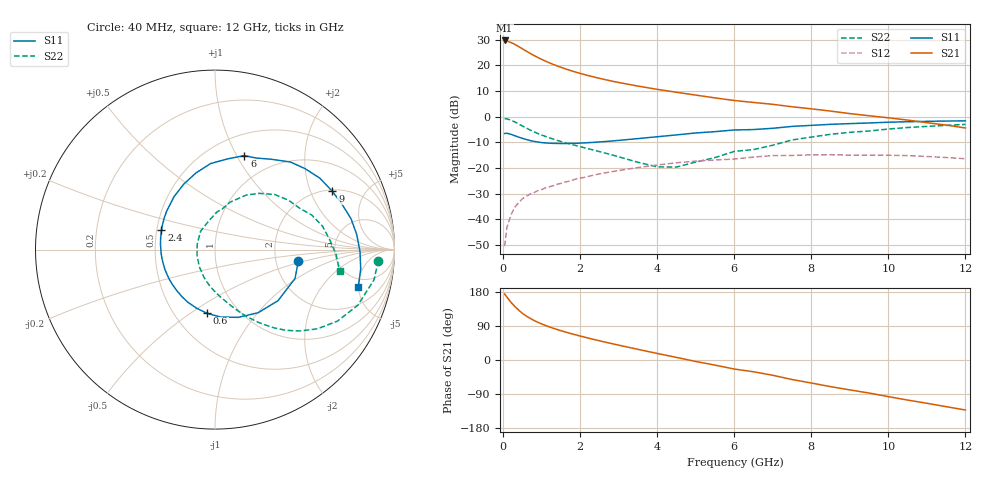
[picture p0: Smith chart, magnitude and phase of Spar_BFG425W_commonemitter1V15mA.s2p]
! Filename: 115bfg425.001
! BFG425W Field C1
! V1=8.654E-001V,V2=1.000E+000V, I1=2.240E-004A, I2=1.501E-002A
# GHz  S  MA  R 50
!  S11  S21  S12  S22
!Freq(GHz)  Mag  Ang  Mag  Ang  Mag  Ang  Mag  Ang
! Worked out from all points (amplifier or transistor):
!   44 points, 40 MHz to 12 GHz, reference 50 ohm
!   highest |S21| = 29.6 dB at 40 MHz (marker M1)
!   |S21| within 3 dB of that: start of sweep to 474.3 MHz
!   unconditionally stable (mu >= 1): 1.434 GHz to end of sweep
!   at 700 MHz: K = 0.69, MSG = 27.4 dB, |S12| = -30.2 dB
!   at 2.4 GHz: K = 1.15, MAG = 16.6 dB, |S12| = -22.6 dB
!   at 12 GHz: K = 1.36, MAG = 2.4 dB, |S12| = -16.4 dB
!   S11 on the Smith chart (normalised r, x): 40 MHz: 2.68, -0.44; 600 MHz: 0.72, -0.58; 2.4 GHz: 0.53, +0.13; 6 GHz: 0.72, +1.08; 9 GHz: 2.07, +2.88; 12 GHz: 3.84, -4.97
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0.04  0.469 -7.9  30.36 174.1  0.003 76.3  0.912 -3.9
0.1  0.474 -19.8  29.61 166.0  0.007 81.6  0.902 -10.7
0.2  0.452 -39.0  27.79 152.8  0.012 74.0  0.854 -21.3
0.3  0.426 -55.7  25.61 141.8  0.017 68.6  0.79 -30.3
0.4  0.399 -71.1  23.21 131.9  0.021 63.9  0.722 -37.7
0.5  0.377 -85.2  20.93 123.3  0.025 60.3  0.657 -43.6
0.6  0.358 -97.0  18.87 116.2  0.028 57.9  0.6 -48.6
0.7  0.342 -107.6  17.07 110.1  0.031 55.9  0.549 -52.7
0.9  0.32 -125.5  14.19 99.6  0.036 53.4  0.47 -59.3
1  0.312 -133.2  13.03 95.2  0.038 52.5  0.438 -62.1
1.2  0.304 -146.4  11.16 87.4  0.043 50.8  0.387 -67.1
1.6  0.299 -168.0  8.59 74.4  0.053 47.8  0.312 -75.8
2.2  0.31 167.4  6.316 58.2  0.068 42.0  0.238 -89.3
2.4  0.317 160.3  5.793 53.2  0.074 39.9  0.218 -94.2
3.5  0.373 127.8  3.924 28.1  0.102 25.5  0.129 -132.9
4.5  0.44 104.0  2.976 6.8  0.126 10.5  0.104 162.0
6  0.549 72.7  2.057 -23.8  0.149 -13.9  0.21 87.0
6.5  0.559 65.8  1.886 -31.0  0.163 -17.8  0.228 80.2
8.5  0.707 34.2  1.28 -70.3  0.181 -53.7  0.452 42.8
9  0.73 26.4  1.144 -78.9  0.178 -61.6  0.494 33.8
10.5  0.794 6.1  0.855 -105.7  0.174 -87.2  0.613 12.4
12  0.825 -14.5  0.6 -131.9  0.151 -115.2  0.705 -9.9
